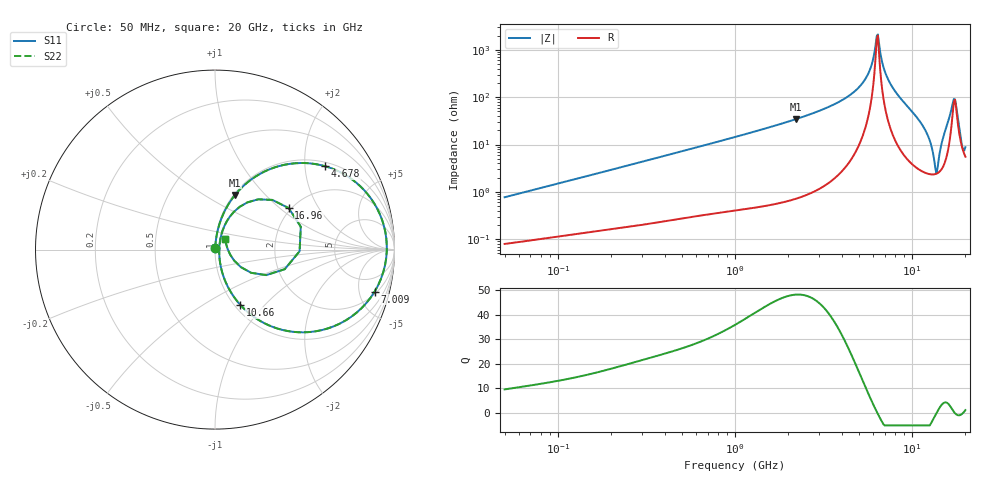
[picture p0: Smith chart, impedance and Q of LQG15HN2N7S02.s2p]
!Murata Part Number: LQG15HN2N7S02
!These Parameters are Measured in Series Mode Connection
!  o--[Z]--o
!Port1  Port2
!  o-------o
!Freq. Start=50[MHz] Stop=20[GHz], 401[Steps]
# Hz S RI R 50
!Freq.(Hz) S11(Real) S11(Imag) S21(Real) S21(Imag) S12(Real) S12(Imag) S22(Real) S22(Imag)
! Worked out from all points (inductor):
!   401 points, 50 MHz to 20 GHz, reference 50 ohm
!   read as one part in series: L = 2.42 nH near 51.52 MHz
!   highest Q = 48.1 at 2.212 GHz (marker M1), where L = 2.48 nH
!   self-resonance near 6.312 GHz
!   S11 on the Smith chart (normalised r, x): 50 MHz: 1.00, +0.02; 4.678 GHz: 1.12, +2.55; 7.009 GHz: 2.29, -6.97; 10.66 GHz: 1.06, -0.74; 16.96 GHz: 1.94, +1.15; 20 GHz: 1.11, +0.14
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5e7  0.000854 0.00765  0.9991 -0.00765  0.9991 -0.00765  0.000854 0.00765
1.364002e8  0.00174 0.0201  0.9983 -0.0201  0.9983 -0.0201  0.00174 0.0201
3.721004e8  0.00515 0.0533  0.9949 -0.0533  0.9949 -0.0533  0.00515 0.0533
1e9  0.0241 0.1402  0.9759 -0.1402  0.9759 -0.1402  0.0241 0.1402
2.211938e9  0.1114 0.3044  0.8886 -0.3044  0.8886 -0.3044  0.1114 0.3044
2.728004e9  0.1751 0.3695  0.8249 -0.3695  0.8249 -0.3695  0.1751 0.3695
3.680849e9  0.3488 0.4631  0.6512 -0.4631  0.6512 -0.4631  0.3488 0.4631
4.677679e9  0.6141 0.4642  0.3859 -0.4642  0.3859 -0.4642  0.6141 0.4642
5.683258e9  0.8867 0.2582  0.1133 -0.2582  0.1133 -0.2582  0.8867 0.2582
6.311513e9  0.9571 0.0245  0.0429 -0.0245  0.0429 -0.0245  0.9571 0.0245
6.503449e9  0.9533 -0.0516  0.0467 0.0516  0.0467 0.0516  0.9533 -0.0516
7.009217e9  0.8891 -0.2346  0.1109 0.2346  0.1109 0.2346  0.8891 -0.2346
7.442007e9  0.7885 -0.3516  0.2115 0.3516  0.2115 0.3516  0.7885 -0.3516
8.644534e9  0.4651 -0.4605  0.5349 0.4605  0.5349 0.4605  0.4651 -0.4605
1.066139e10  0.1409 -0.3076  0.8591 0.3076  0.8591 0.3076  0.1409 -0.3076
1.220001e10  0.0475 -0.1502  0.9525 0.1502  0.9525 0.1502  0.0475 -0.1502
1.375312e10  0.0237 0.00168  0.9763 -0.00168  0.9763 -0.00168  0.0237 0.00168
1.573793e10  0.1063 0.2114  0.8937 -0.2114  0.8937 -0.2114  0.1063 0.2114
1.696185e10  0.4103 0.2317  0.5897 -0.2317  0.5897 -0.2317  0.4103 0.2317
1.800918e10  0.2852 -0.1421  0.7148 0.1421  0.7148 0.1421  0.2852 -0.1421
1.912117e10  0.0838 -0.0265  0.9162 0.0265  0.9162 0.0265  0.0838 -0.0265
2e10  0.0565 0.0612  0.9435 -0.0612  0.9435 -0.0612  0.0565 0.0612
